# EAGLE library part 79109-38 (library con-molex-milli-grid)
RECEPTACAL
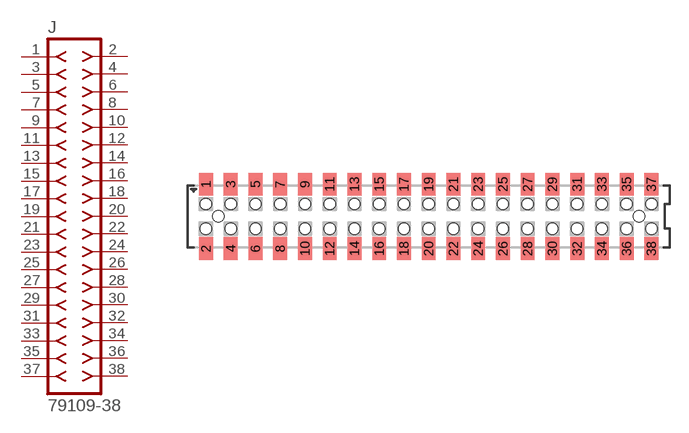
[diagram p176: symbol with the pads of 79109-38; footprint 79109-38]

Designator prefix J

## 79109-38  [79109-38]
1  1  pas
2  2  pas
3  3  pas
4  4  pas
5  5  pas
6  6  pas
7  7  pas
8  8  pas
9  9  pas
10  10  pas
11  11  pas
12  12  pas
13  13  pas
14  14  pas
15  15  pas
16  16  pas
17  17  pas
18  18  pas
19  19  pas
20  20  pas
21  21  pas
22  22  pas
23  23  pas
24  24  pas
25  25  pas
26  26  pas
27  27  pas
28  28  pas
29  29  pas
30  30  pas
31  31  pas
32  32  pas
33  33  pas
34  34  pas
35  35  pas
36  36  pas
37  37  pas
38  38  pas

## Footprint 79109-38 (pad centres in mm)
RECEPTACAL SMD Dual Row, Vertical, Pass-Thru
smd 1.12 x 1.83: 1 -18,2.6; 2 -18,-2.6; 3 -16,2.6; 4 -16,-2.6; 5 -14,2.6; 6 -14,-2.6; 7 -12,2.6; 8 -12,-2.6; 9 -10,2.6; 10 -10,-2.6; 11 -8,2.6; 12 -8,-2.6; 13 -6,2.6; 14 -6,-2.6; 15 -4,2.6; 16 -4,-2.6; 17 -2,2.6; 18 -2,-2.6; 19 0,2.6; 20 0,-2.6; 21 2,2.6; 22 2,-2.6; 23 4,2.6; 24 4,-2.6; 25 6,2.6; 26 6,-2.6; 27 8,2.6; 28 8,-2.6; 29 10,2.6; 30 10,-2.6; 31 12,2.6; 32 12,-2.6; 33 14,2.6; 34 14,-2.6; 35 16,2.6; 36 16,-2.6; 37 18,2.6; 38 18,-2.6
hole 0.914 at -17,0
hole 0.914 at -18,1
hole 0.914 at -18,-1
hole 0.914 at -16,-1
hole 0.914 at -16,1
hole 0.914 at -14,-1
hole 0.914 at -14,1
hole 0.914 at 17,0
hole 0.914 at -12,1
hole 0.914 at -12,-1
hole 0.914 at -10,1
hole 0.914 at -10,-1
hole 0.914 at -8,1
hole 0.914 at -8,-1
hole 0.914 at -6,1
hole 0.914 at -6,-1
hole 0.914 at -4,-1
hole 0.914 at -4,1
hole 0.914 at -2,1
hole 0.914 at -2,-1
hole 0.914 at 0,1
hole 0.914 at 0,-1
hole 0.914 at 2,1
hole 0.914 at 2,-1
hole 0.914 at 4,-1
hole 0.914 at 4,1
hole 0.914 at 6,1
hole 0.914 at 8,1
hole 0.914 at 10,1
hole 0.914 at 6,-1
hole 0.914 at 8,-1
hole 0.914 at 10,-1
hole 0.914 at 12,-1
hole 0.914 at 14,-1
hole 0.914 at 16,-1
hole 0.914 at 18,-1
hole 0.914 at 12,1
hole 0.914 at 14,1
hole 0.914 at 16,1
hole 0.914 at 18,1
